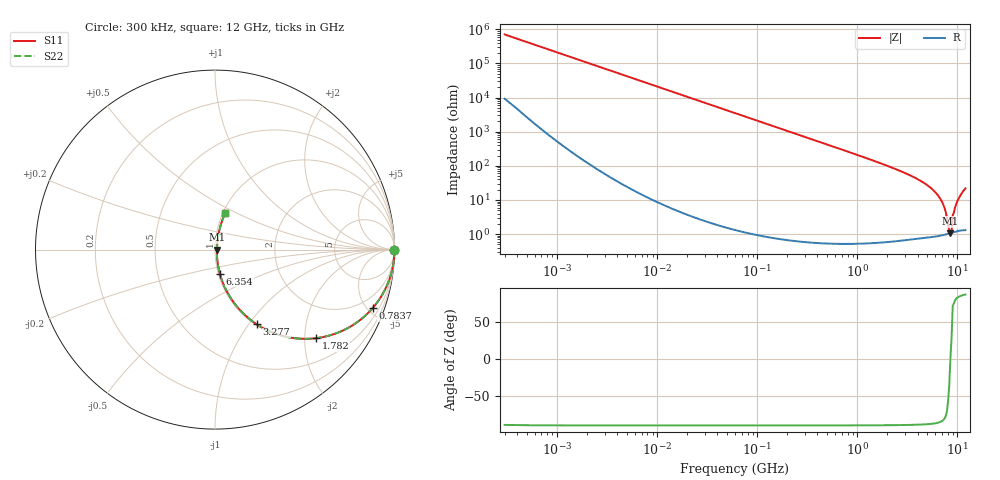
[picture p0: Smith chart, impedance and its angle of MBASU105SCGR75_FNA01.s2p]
! MBASU105SCGR75_FNA01  S-PARAMETER MODEL  ( Standard Model )
! Model Generated by TAIYO YUDEN Corporation (http://www.ty-top.com)
! Version 1.0
! TAIYO YUDEN Control No. 230609
! Copyright(c) 2023 TAIYO YUDEN CO.,LTD. All Rights Reserved.
! Product Description (link to TY-COMPAS)
! https://ds.yuden.co.jp/TYCOMPAS/or/detail?pn=MBASU105SCGR75CFNA01&u=M
! Products Name : Multilayer Ceramic Capacitors
! Characteristics :
!  Capacitance : 0.75 [pF] , Rated Voltage : 50 [V] , TCC : CG / C0G
!  Case Size : 1.0 x 0.5 / 0.039 x 0.02 [mm/inch] , Thickness : 0.5 / 0.02 [mm/inch]
!  (Conditions: Temperature = 25 [degC] , DC Bias Voltage = 0 [V])
! External Node Assignments :
!  1  o---| |---o  2
! GND o---------o GND
! Frequency Range : 0.3MHz  -  12000MHz  [ 401 STEP ]
# MHZ S RI R 50
! Freq[MHz].  S11 Real  S11 Imag  S21 Real  S21 Imag  S12 Real  S12 Imag  S22 Real  S22 Imag
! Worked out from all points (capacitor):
!   401 points, 300 kHz to 12 GHz, reference 50 ohm
!   read as one part in series: C = 750 fF near 316.3 kHz
!   lowest |Z| = 1.07 ohm at 8.504 GHz (marker M1)
!   series resonance near 8.499 GHz, so ESL is about 470 pH
!   S11 on the Smith chart (normalised r, x): 300 kHz: open; 783.7 MHz: 1.01, -5.37; 1.782 GHz: 1.01, -2.27; 3.277 GHz: 1.01, -1.09; 6.354 GHz: 1.02, -0.28; 12 GHz: 1.03, +0.44
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0.3  1 -0.000141  1.88e-06 0.000141  1.88e-06 0.000141  1 -0.000141
1.769972  1 -0.000834  1.79e-06 0.000834  1.79e-06 0.000834  1 -0.000834
10.44266  1 -0.00492  2.62e-05 0.00492  2.62e-05 0.00492  1 -0.00492
60  0.9992 -0.0283  0.000809 0.0283  0.000809 0.0283  0.9992 -0.0283
164.1901  0.994 -0.0769  0.006 0.0769  0.006 0.0769  0.994 -0.0769
353.9943  0.9727 -0.1625  0.0273 0.1625  0.0273 0.1625  0.9727 -0.1625
783.7017  0.8776 -0.3268  0.1224 0.3268  0.1224 0.3268  0.8776 -0.3268
1166.079  0.7603 -0.4254  0.2397 0.4254  0.2397 0.4254  0.7603 -0.4254
1781.601  0.5633 -0.4935  0.4367 0.4935  0.4367 0.4935  0.5633 -0.4935
2088.533  0.4756 -0.4963  0.5244 0.4963  0.5244 0.4963  0.4756 -0.4963
3276.641  0.2332 -0.4166  0.7668 0.4166  0.7668 0.4166  0.2332 -0.4166
4875.354  0.0816 -0.2603  0.9184 0.2603  0.9184 0.2603  0.0816 -0.2603
6354.153  0.0271 -0.134  0.9729 0.134  0.9729 0.134  0.0271 -0.134
7254.098  0.014 -0.0682  0.986 0.0682  0.986 0.0682  0.014 -0.0682
8281.503  0.0104 -0.00737  0.9896 0.00737  0.9896 0.00737  0.0104 -0.00737
8503.825  0.0106 0.000163  0.9894 -0.000163  0.9894 -0.000163  0.0106 0.000163
8732.115  0.0108 0.00573  0.9892 -0.00573  0.9892 -0.00573  0.0108 0.00573
8966.534  0.0121 0.0325  0.9879 -0.0325  0.9879 -0.0325  0.0121 0.0325
9454.42  0.015 0.058  0.985 -0.058  0.985 -0.058  0.015 0.058
9968.853  0.02 0.0881  0.98 -0.0881  0.98 -0.0881  0.02 0.0881
11083.22  0.0368 0.1522  0.9632 -0.1522  0.9632 -0.1522  0.0368 0.1522
12000  0.0568 0.2035  0.9432 -0.2035  0.9432 -0.2035  0.0568 0.2035
